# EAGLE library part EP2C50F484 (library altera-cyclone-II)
EP2C50F484 Auto generated by make-symbol-device-package-bsdl.ulp Rev. 19 Tip: Use split-device-symbol.ulp to generate a Device with multiple small symbols! Read HELP. Source: EP2C50F484.BSD
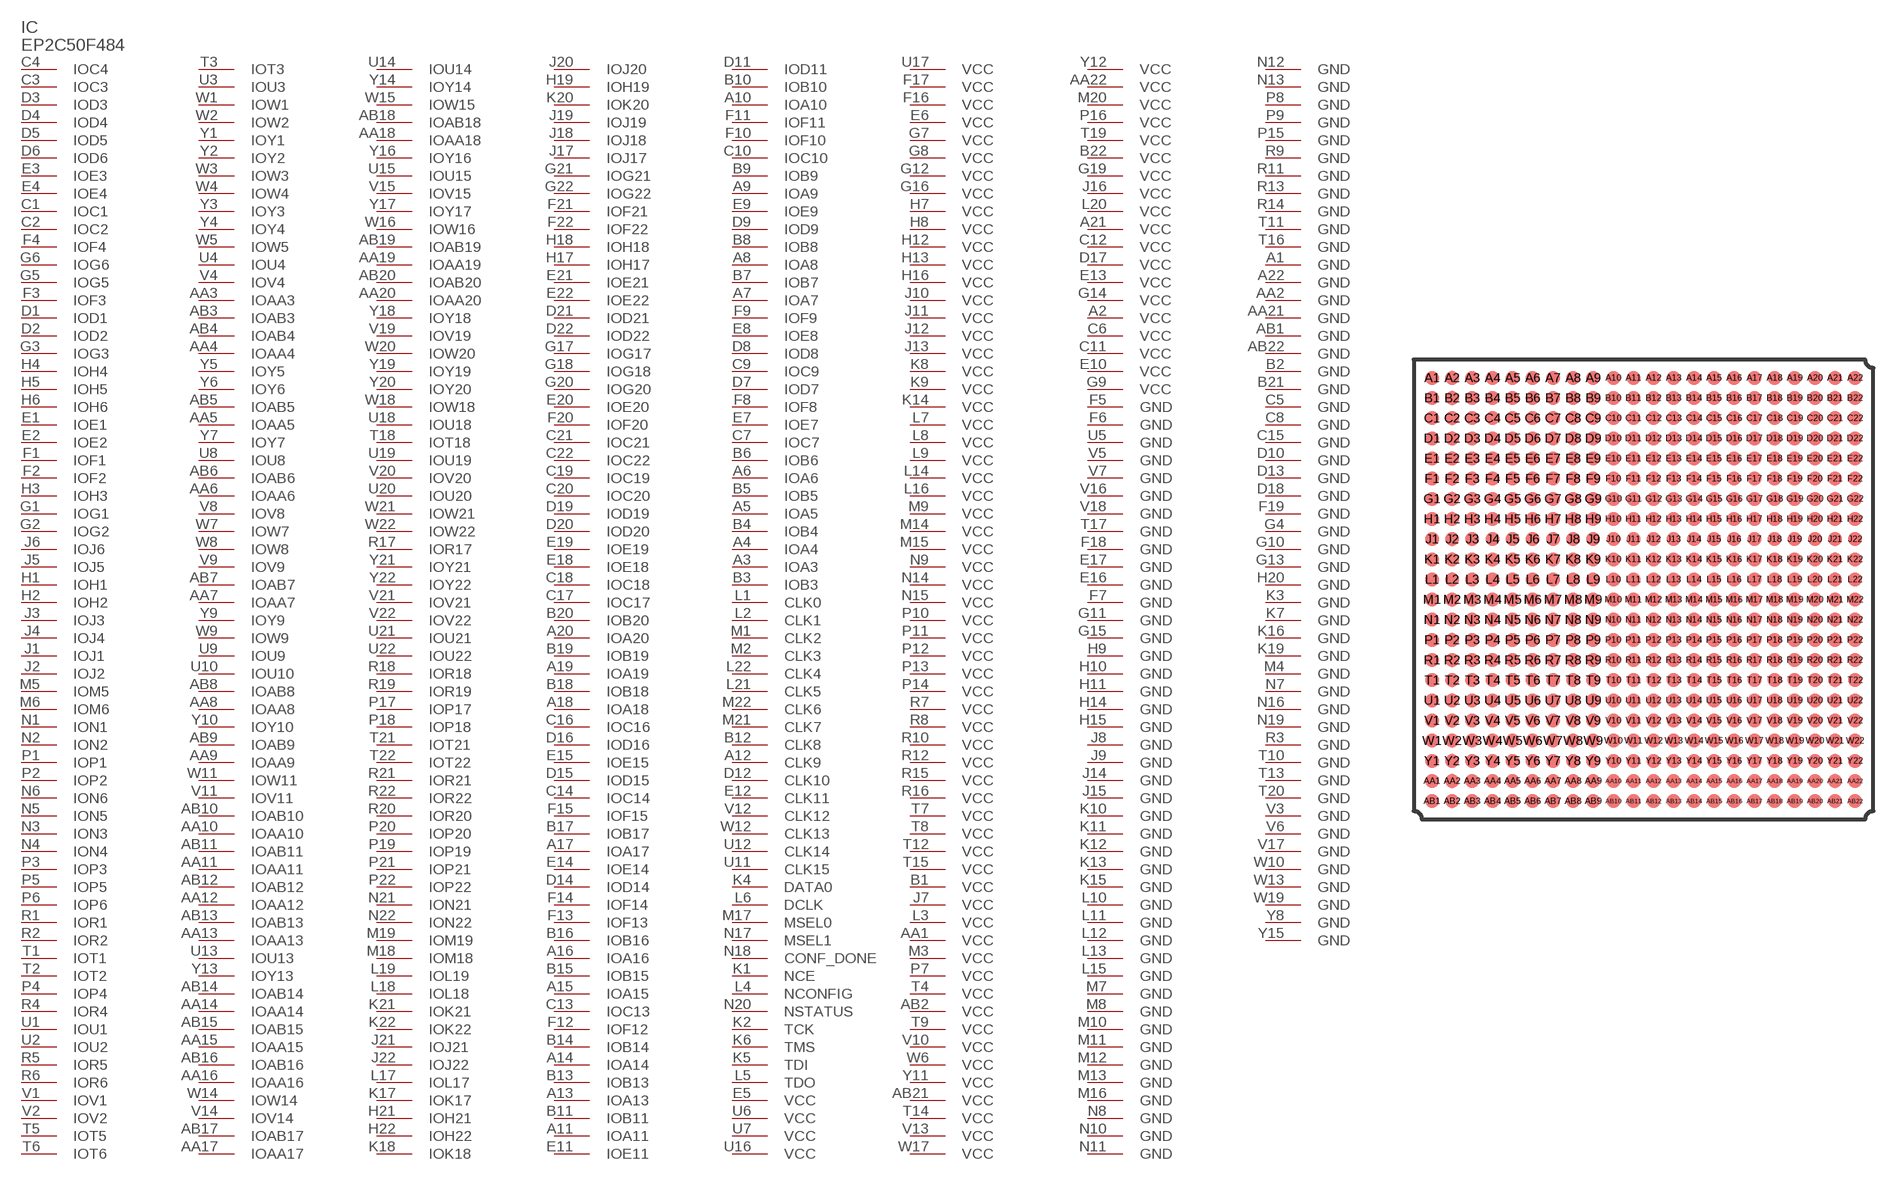
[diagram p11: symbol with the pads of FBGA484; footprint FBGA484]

Designator prefix IC

## EP2C50F484 (MPN: EP2C50F484C8N; OC_FARNELL: 1549358; OC_NEWARK: 51R0569)  [FBGA484]
A1  GND  pwr
A2  VCC  pwr
A3  IOA3
A4  IOA4
A5  IOA5
A6  IOA6
A7  IOA7
A8  IOA8
A9  IOA9
A10  IOA10
A11  IOA11
A12  CLK9
A13  IOA13
A14  IOA14
A15  IOA15
A16  IOA16
A17  IOA17
A18  IOA18
A19  IOA19
A20  IOA20
A21  VCC  pwr
A22  GND  pwr
AA1  VCC  pwr
AA2  GND  pwr
AA3  IOAA3
AA4  IOAA4
AA5  IOAA5
AA6  IOAA6
AA7  IOAA7
AA8  IOAA8
AA9  IOAA9
AA10  IOAA10
AA11  IOAA11
AA12  IOAA12
AA13  IOAA13
AA14  IOAA14
AA15  IOAA15
AA16  IOAA16
AA17  IOAA17
AA18  IOAA18
AA19  IOAA19
AA20  IOAA20
AA21  GND  pwr
AA22  VCC  pwr
AB1  GND  pwr
AB2  VCC  pwr
AB3  IOAB3
AB4  IOAB4
AB5  IOAB5
AB6  IOAB6
AB7  IOAB7
AB8  IOAB8
AB9  IOAB9
AB10  IOAB10
AB11  IOAB11
AB12  IOAB12
AB13  IOAB13
AB14  IOAB14
AB15  IOAB15
AB16  IOAB16
AB17  IOAB17
AB18  IOAB18
AB19  IOAB19
AB20  IOAB20
AB21  VCC  pwr
AB22  GND  pwr
B1  VCC  pwr
B2  GND  pwr
B3  IOB3
B4  IOB4
B5  IOB5
B6  IOB6
B7  IOB7
B8  IOB8
B9  IOB9
B10  IOB10
B11  IOB11
B12  CLK8
B13  IOB13
B14  IOB14
B15  IOB15
B16  IOB16
B17  IOB17
B18  IOB18
B19  IOB19
B20  IOB20
B21  GND  pwr
B22  VCC  pwr
C1  IOC1
C2  IOC2
C3  IOC3  out
C4  IOC4  out
C5  GND  pwr
C6  VCC  pwr
C7  IOC7
C8  GND  pwr
C9  IOC9
C10  IOC10
C11  VCC  pwr
C12  VCC  pwr
C13  IOC13
C14  IOC14
C15  GND  pwr
C16  IOC16
C17  IOC17
C18  IOC18
C19  IOC19
C20  IOC20
C21  IOC21
C22  IOC22
D1  IOD1
D2  IOD2
D3  IOD3
D4  IOD4
D5  IOD5
D6  IOD6
D7  IOD7
D8  IOD8
D9  IOD9
D10  GND  pwr
D11  IOD11
D12  CLK10
D13  GND  pwr
D14  IOD14
D15  IOD15
D16  IOD16
D17  VCC  pwr
D18  GND  pwr
D19  IOD19
D20  IOD20
D21  IOD21
D22  IOD22
E1  IOE1
E2  IOE2
E3  IOE3
E4  IOE4
E5  VCC  pwr
E6  VCC  pwr
E7  IOE7
E8  IOE8
E9  IOE9
E10  VCC  pwr
E11  IOE11
E12  CLK11
E13  VCC  pwr
E14  IOE14
E15  IOE15
E16  GND  pwr
E17  GND  pwr
E18  IOE18
E19  IOE19
E20  IOE20
E21  IOE21
E22  IOE22
F1  IOF1
F2  IOF2
F3  IOF3
F4  IOF4
F5  GND  pwr
F6  GND  pwr
F7  GND  pwr
F8  IOF8
F9  IOF9
F10  IOF10
F11  IOF11
F12  IOF12
F13  IOF13
F14  IOF14
F15  IOF15
F16  VCC  pwr
F17  VCC  pwr
F18  GND  pwr
F19  GND  pwr
F20  IOF20
F21  IOF21
F22  IOF22
G1  IOG1
G2  IOG2
G3  IOG3
G4  GND  pwr
G5  IOG5
G6  IOG6
G7  VCC  pwr
G8  VCC  pwr
G9  VCC  pwr
G10  GND  pwr
G11  GND  pwr
G12  VCC  pwr
G13  GND  pwr
G14  VCC  pwr
G15  GND  pwr
G16  VCC  pwr
G17  IOG17
G18  IOG18
G19  VCC  pwr
G20  IOG20
G21  IOG21
G22  IOG22
H1  IOH1
H2  IOH2
H3  IOH3
H4  IOH4
H5  IOH5
H6  IOH6
H7  VCC  pwr
H8  VCC  pwr
H9  GND  pwr
H10  GND  pwr
H11  GND  pwr
H12  VCC  pwr
H13  VCC  pwr
H14  GND  pwr
H15  GND  pwr
H16  VCC  pwr
H17  IOH17
H18  IOH18
H19  IOH19
H20  GND  pwr
H21  IOH21
H22  IOH22
J1  IOJ1
J2  IOJ2
J3  IOJ3
J4  IOJ4
J5  IOJ5
J6  IOJ6
J7  VCC  pwr
J8  GND  pwr
J9  GND  pwr
J10  VCC  pwr
J11  VCC  pwr
J12  VCC  pwr
J13  VCC  pwr
J14  GND  pwr
J15  GND  pwr
J16  VCC  pwr
J17  IOJ17
J18  IOJ18
J19  IOJ19
J20  IOJ20
J21  IOJ21
J22  IOJ22
K1  NCE  in
K2  TCK  in
K3  GND  pwr
K4  DATA0
K5  TDI  in
K6  TMS  in
K7  GND  pwr
K8  VCC  pwr
K9  VCC  pwr
K10  GND  pwr
K11  GND  pwr
K12  GND  pwr
K13  GND  pwr
K14  VCC  pwr
K15  GND  pwr
K16  GND  pwr
K17  IOK17
K18  IOK18
K19  GND  pwr
K20  IOK20
K21  IOK21
K22  IOK22
L1  CLK0
L2  CLK1
L3  VCC  pwr
L4  NCONFIG  in
L5  TDO  out
L6  DCLK
L7  VCC  pwr
L8  VCC  pwr
L9  VCC  pwr
L10  GND  pwr
L11  GND  pwr
L12  GND  pwr
L13  GND  pwr
L14  VCC  pwr
L15  GND  pwr
L16  VCC  pwr
L17  IOL17
L18  IOL18
L19  IOL19
L20  VCC  pwr
L21  CLK5
L22  CLK4
M1  CLK2
M2  CLK3
M3  VCC  pwr
M4  GND  pwr
M5  IOM5
M6  IOM6
M7  GND  pwr
M8  GND  pwr
M9  VCC  pwr
M10  GND  pwr
M11  GND  pwr
M12  GND  pwr
M13  GND  pwr
M14  VCC  pwr
M15  VCC  pwr
M16  GND  pwr
M17  MSEL0  in
M18  IOM18
M19  IOM19
M20  VCC  pwr
M21  CLK7
M22  CLK6
N1  ION1
N2  ION2
N3  ION3
N4  ION4
N5  ION5
N6  ION6
N7  GND  pwr
N8  GND  pwr
N9  VCC  pwr
N10  GND  pwr
N11  GND  pwr
N12  GND  pwr
N13  GND  pwr
N14  VCC  pwr
N15  VCC  pwr
N16  GND  pwr
N17  MSEL1  in
N18  CONF_DONE  in
N19  GND  pwr
N20  NSTATUS  in
N21  ION21
N22  ION22
P1  IOP1
P2  IOP2
P3  IOP3
P4  IOP4
P5  IOP5
P6  IOP6
P7  VCC  pwr
P8  GND  pwr
P9  GND  pwr
P10  VCC  pwr
P11  VCC  pwr
P12  VCC  pwr
P13  VCC  pwr
P14  VCC  pwr
P15  GND  pwr
P16  VCC  pwr
P17  IOP17
P18  IOP18
P19  IOP19
P20  IOP20
P21  IOP21
P22  IOP22
R1  IOR1
R2  IOR2
R3  GND  pwr
R4  IOR4
R5  IOR5
R6  IOR6
R7  VCC  pwr
R8  VCC  pwr
R9  GND  pwr
R10  VCC  pwr
R11  GND  pwr
R12  VCC  pwr
R13  GND  pwr
R14  GND  pwr
R15  VCC  pwr
R16  VCC  pwr
R17  IOR17
R18  IOR18
R19  IOR19
R20  IOR20
R21  IOR21
R22  IOR22
T1  IOT1
T2  IOT2
T3  IOT3
T4  VCC  pwr
T5  IOT5
T6  IOT6
T7  VCC  pwr
T8  VCC  pwr
T9  VCC  pwr
T10  GND  pwr
T11  GND  pwr
T12  VCC  pwr
T13  GND  pwr
T14  VCC  pwr
T15  VCC  pwr
T16  GND  pwr
T17  GND  pwr
T18  IOT18
T19  VCC  pwr
T20  GND  pwr
T21  IOT21
T22  IOT22
U1  IOU1
U2  IOU2
U3  IOU3
U4  IOU4
U5  GND  pwr
U6  VCC  pwr
U7  VCC  pwr
U8  IOU8
U9  IOU9
U10  IOU10
U11  CLK15
U12  CLK14
U13  IOU13
U14  IOU14
U15  IOU15
U16  VCC  pwr
U17  VCC  pwr
U18  IOU18
U19  IOU19
U20  IOU20
U21  IOU21
U22  IOU22
V1  IOV1
V2  IOV2
V3  GND  pwr
V4  IOV4
V5  GND  pwr
V6  GND  pwr
V7  GND  pwr
V8  IOV8
V9  IOV9
V10  VCC  pwr
V11  IOV11
V12  CLK12
V13  VCC  pwr
V14  IOV14
V15  IOV15
V16  GND  pwr
V17  GND  pwr
V18  GND  pwr
V19  IOV19
V20  IOV20
V21  IOV21
V22  IOV22
W1  IOW1
W2  IOW2
W3  IOW3
W4  IOW4
W5  IOW5
W6  VCC  pwr
W7  IOW7
W8  IOW8
W9  IOW9
W10  GND  pwr
W11  IOW11
W12  CLK13
W13  GND  pwr
W14  IOW14
W15  IOW15
W16  IOW16
W17  VCC  pwr
W18  IOW18
W19  GND  pwr
W20  IOW20
W21  IOW21
W22  IOW22
Y1  IOY1
Y2  IOY2
Y3  IOY3
Y4  IOY4
Y5  IOY5
Y6  IOY6
Y7  IOY7
Y8  GND  pwr
Y9  IOY9
Y10  IOY10
Y11  VCC  pwr
Y12  VCC  pwr
Y13  IOY13
Y14  IOY14
Y15  GND  pwr
Y16  IOY16
Y17  IOY17
Y18  IOY18
Y19  IOY19
Y20  IOY20
Y21  IOY21
Y22  IOY22

## Footprint FBGA484 (pad centres in mm)
EP2C15AF484 Auto generated by make-symbol-device-package-bsdl.ulp Rev. 18 Source: EP2C15AF484.BSD www.altera.com .. cyc2_cii51015.pdf
smd 0.7 x 0.7: A1 -10.5,10.5; A2 -9.5,10.5; A3 -8.5,10.5; A4 -7.5,10.5; A5 -6.5,10.5; A6 -5.5,10.5; A7 -4.5,10.5; A8 -3.5,10.5; A9 -2.5,10.5; A10 -1.5,10.5; A11 -0.5,10.5; A12 0.5,10.5; A13 1.5,10.5; A14 2.5,10.5; A15 3.5,10.5; A16 4.5,10.5; A17 5.5,10.5; A18 6.5,10.5; A19 7.5,10.5; A20 8.5,10.5; A21 9.5,10.5; A22 10.5,10.5; AA1 -10.5,-9.5; AA2 -9.5,-9.5; AA3 -8.5,-9.5; AA4 -7.5,-9.5; AA5 -6.5,-9.5; AA6 -5.5,-9.5; AA7 -4.5,-9.5; AA8 -3.5,-9.5; AA9 -2.5,-9.5; AA10 -1.5,-9.5; AA11 -0.5,-9.5; AA12 0.5,-9.5; AA13 1.5,-9.5; AA14 2.5,-9.5; AA15 3.5,-9.5; AA16 4.5,-9.5; AA17 5.5,-9.5; AA18 6.5,-9.5; AA19 7.5,-9.5; AA20 8.5,-9.5; AA21 9.5,-9.5; AA22 10.5,-9.5; AB1 -10.5,-10.5; AB2 -9.5,-10.5; AB3 -8.5,-10.5; AB4 -7.5,-10.5; AB5 -6.5,-10.5; AB6 -5.5,-10.5; AB7 -4.5,-10.5; AB8 -3.5,-10.5; AB9 -2.5,-10.5; AB10 -1.5,-10.5; AB11 -0.5,-10.5; AB12 0.5,-10.5; AB13 1.5,-10.5; AB14 2.5,-10.5; AB15 3.5,-10.5; AB16 4.5,-10.5; AB17 5.5,-10.5; AB18 6.5,-10.5; AB19 7.5,-10.5; AB20 8.5,-10.5; AB21 9.5,-10.5; AB22 10.5,-10.5; B1 -10.5,9.5; B2 -9.5,9.5; B3 -8.5,9.5; B4 -7.5,9.5; B5 -6.5,9.5; B6 -5.5,9.5; B7 -4.5,9.5; B8 -3.5,9.5; B9 -2.5,9.5; B10 -1.5,9.5; B11 -0.5,9.5; B12 0.5,9.5; B13 1.5,9.5; B14 2.5,9.5; B15 3.5,9.5; B16 4.5,9.5; B17 5.5,9.5; B18 6.5,9.5; B19 7.5,9.5; B20 8.5,9.5; B21 9.5,9.5; B22 10.5,9.5; C1 -10.5,8.5; C2 -9.5,8.5; C3 -8.5,8.5; C4 -7.5,8.5; C5 -6.5,8.5; C6 -5.5,8.5; C7 -4.5,8.5; C8 -3.5,8.5; C9 -2.5,8.5; C10 -1.5,8.5; C11 -0.5,8.5; C12 0.5,8.5; C13 1.5,8.5; C14 2.5,8.5; C15 3.5,8.5; C16 4.5,8.5; C17 5.5,8.5; C18 6.5,8.5; C19 7.5,8.5; C20 8.5,8.5; C21 9.5,8.5; C22 10.5,8.5; D1 -10.5,7.5; D2 -9.5,7.5; D3 -8.5,7.5; D4 -7.5,7.5; D5 -6.5,7.5; D6 -5.5,7.5; D7 -4.5,7.5; D8 -3.5,7.5; D9 -2.5,7.5; D10 -1.5,7.5; D11 -0.5,7.5; D12 0.5,7.5; D13 1.5,7.5; D14 2.5,7.5; D15 3.5,7.5; D16 4.5,7.5; D17 5.5,7.5; D18 6.5,7.5; D19 7.5,7.5; D20 8.5,7.5; D21 9.5,7.5; D22 10.5,7.5; E1 -10.5,6.5; E2 -9.5,6.5; E3 -8.5,6.5; E4 -7.5,6.5; E5 -6.5,6.5; E6 -5.5,6.5; E7 -4.5,6.5; E8 -3.5,6.5; E9 -2.5,6.5; E10 -1.5,6.5; E11 -0.5,6.5; E12 0.5,6.5; E13 1.5,6.5; E14 2.5,6.5; E15 3.5,6.5; E16 4.5,6.5; E17 5.5,6.5; E18 6.5,6.5; E19 7.5,6.5; E20 8.5,6.5; E21 9.5,6.5; E22 10.5,6.5; F1 -10.5,5.5; F2 -9.5,5.5; F3 -8.5,5.5; F4 -7.5,5.5; F5 -6.5,5.5; F6 -5.5,5.5; F7 -4.5,5.5; F8 -3.5,5.5; F9 -2.5,5.5; F10 -1.5,5.5; F11 -0.5,5.5; F12 0.5,5.5; F13 1.5,5.5; F14 2.5,5.5; F15 3.5,5.5; F16 4.5,5.5; F17 5.5,5.5; F18 6.5,5.5; F19 7.5,5.5; F20 8.5,5.5; F21 9.5,5.5; F22 10.5,5.5; G1 -10.5,4.5; G2 -9.5,4.5; G3 -8.5,4.5; G4 -7.5,4.5; G5 -6.5,4.5; G6 -5.5,4.5; G7 -4.5,4.5; G8 -3.5,4.5; G9 -2.5,4.5; G10 -1.5,4.5; G11 -0.5,4.5; G12 0.5,4.5; G13 1.5,4.5; G14 2.5,4.5; G15 3.5,4.5; G16 4.5,4.5; G17 5.5,4.5; G18 6.5,4.5; G19 7.5,4.5; G20 8.5,4.5; G21 9.5,4.5; G22 10.5,4.5; H1 -10.5,3.5; H2 -9.5,3.5; H3 -8.5,3.5; H4 -7.5,3.5; H5 -6.5,3.5; H6 -5.5,3.5; H7 -4.5,3.5; H8 -3.5,3.5; H9 -2.5,3.5; H10 -1.5,3.5; H11 -0.5,3.5; H12 0.5,3.5; H13 1.5,3.5; H14 2.5,3.5; H15 3.5,3.5; H16 4.5,3.5; H17 5.5,3.5; H18 6.5,3.5; H19 7.5,3.5; H20 8.5,3.5; H21 9.5,3.5; H22 10.5,3.5; J1 -10.5,2.5; J2 -9.5,2.5; J3 -8.5,2.5; J4 -7.5,2.5; J5 -6.5,2.5; J6 -5.5,2.5; J7 -4.5,2.5; J8 -3.5,2.5; J9 -2.5,2.5; J10 -1.5,2.5; J11 -0.5,2.5; J12 0.5,2.5; J13 1.5,2.5; J14 2.5,2.5; J15 3.5,2.5; J16 4.5,2.5; J17 5.5,2.5; J18 6.5,2.5; J19 7.5,2.5; J20 8.5,2.5; J21 9.5,2.5; J22 10.5,2.5; K1 -10.5,1.5; K2 -9.5,1.5; K3 -8.5,1.5; K4 -7.5,1.5; K5 -6.5,1.5; K6 -5.5,1.5; K7 -4.5,1.5; K8 -3.5,1.5; K9 -2.5,1.5; K10 -1.5,1.5; K11 -0.5,1.5; K12 0.5,1.5; K13 1.5,1.5; K14 2.5,1.5; K15 3.5,1.5; K16 4.5,1.5; K17 5.5,1.5; K18 6.5,1.5; K19 7.5,1.5; K20 8.5,1.5; K21 9.5,1.5; K22 10.5,1.5; L1 -10.5,0.5; L2 -9.5,0.5; L3 -8.5,0.5; L4 -7.5,0.5; L5 -6.5,0.5; L6 -5.5,0.5; L7 -4.5,0.5; L8 -3.5,0.5; L9 -2.5,0.5; L10 -1.5,0.5; L11 -0.5,0.5; L12 0.5,0.5; L13 1.5,0.5; L14 2.5,0.5; L15 3.5,0.5; L16 4.5,0.5; L17 5.5,0.5; L18 6.5,0.5; L19 7.5,0.5; L20 8.5,0.5; L21 9.5,0.5; L22 10.5,0.5; M1 -10.5,-0.5; M2 -9.5,-0.5; M3 -8.5,-0.5; M4 -7.5,-0.5; M5 -6.5,-0.5; M6 -5.5,-0.5; M7 -4.5,-0.5; M8 -3.5,-0.5; M9 -2.5,-0.5; M10 -1.5,-0.5; M11 -0.5,-0.5; M12 0.5,-0.5; M13 1.5,-0.5; M14 2.5,-0.5; M15 3.5,-0.5; M16 4.5,-0.5; M17 5.5,-0.5; M18 6.5,-0.5; M19 7.5,-0.5; M20 8.5,-0.5; M21 9.5,-0.5; M22 10.5,-0.5; N1 -10.5,-1.5; N2 -9.5,-1.5; N3 -8.5,-1.5; N4 -7.5,-1.5; N5 -6.5,-1.5; N6 -5.5,-1.5; N7 -4.5,-1.5; N8 -3.5,-1.5; N9 -2.5,-1.5; N10 -1.5,-1.5; N11 -0.5,-1.5; N12 0.5,-1.5; N13 1.5,-1.5; N14 2.5,-1.5; N15 3.5,-1.5; N16 4.5,-1.5; N17 5.5,-1.5; N18 6.5,-1.5; N19 7.5,-1.5; N20 8.5,-1.5; N21 9.5,-1.5; N22 10.5,-1.5; P1 -10.5,-2.5; P2 -9.5,-2.5; P3 -8.5,-2.5; P4 -7.5,-2.5; P5 -6.5,-2.5; P6 -5.5,-2.5; P7 -4.5,-2.5; P8 -3.5,-2.5; P9 -2.5,-2.5; P10 -1.5,-2.5; P11 -0.5,-2.5; P12 0.5,-2.5; P13 1.5,-2.5; P14 2.5,-2.5; P15 3.5,-2.5; P16 4.5,-2.5; P17 5.5,-2.5; P18 6.5,-2.5; P19 7.5,-2.5; P20 8.5,-2.5; P21 9.5,-2.5; P22 10.5,-2.5; R1 -10.5,-3.5; R2 -9.5,-3.5; R3 -8.5,-3.5; R4 -7.5,-3.5; R5 -6.5,-3.5; R6 -5.5,-3.5; R7 -4.5,-3.5; R8 -3.5,-3.5; R9 -2.5,-3.5; R10 -1.5,-3.5; R11 -0.5,-3.5; R12 0.5,-3.5; R13 1.5,-3.5; R14 2.5,-3.5; R15 3.5,-3.5; R16 4.5,-3.5; R17 5.5,-3.5; R18 6.5,-3.5; R19 7.5,-3.5; R20 8.5,-3.5; R21 9.5,-3.5; R22 10.5,-3.5; T1 -10.5,-4.5; T2 -9.5,-4.5; T3 -8.5,-4.5; T4 -7.5,-4.5; T5 -6.5,-4.5; T6 -5.5,-4.5; T7 -4.5,-4.5; T8 -3.5,-4.5; T9 -2.5,-4.5; T10 -1.5,-4.5; T11 -0.5,-4.5; T12 0.5,-4.5; T13 1.5,-4.5; T14 2.5,-4.5; T15 3.5,-4.5; T16 4.5,-4.5; T17 5.5,-4.5; T18 6.5,-4.5; T19 7.5,-4.5; T20 8.5,-4.5; T21 9.5,-4.5; T22 10.5,-4.5; U1 -10.5,-5.5; U2 -9.5,-5.5; U3 -8.5,-5.5; U4 -7.5,-5.5; U5 -6.5,-5.5; U6 -5.5,-5.5; U7 -4.5,-5.5; U8 -3.5,-5.5; U9 -2.5,-5.5; U10 -1.5,-5.5; U11 -0.5,-5.5; U12 0.5,-5.5; U13 1.5,-5.5; U14 2.5,-5.5; U15 3.5,-5.5; U16 4.5,-5.5; U17 5.5,-5.5; U18 6.5,-5.5; U19 7.5,-5.5; U20 8.5,-5.5; U21 9.5,-5.5; U22 10.5,-5.5; V1 -10.5,-6.5; V2 -9.5,-6.5; V3 -8.5,-6.5; V4 -7.5,-6.5; V5 -6.5,-6.5; V6 -5.5,-6.5; V7 -4.5,-6.5; V8 -3.5,-6.5; V9 -2.5,-6.5; V10 -1.5,-6.5; V11 -0.5,-6.5; V12 0.5,-6.5; V13 1.5,-6.5; V14 2.5,-6.5; V15 3.5,-6.5; V16 4.5,-6.5; V17 5.5,-6.5; V18 6.5,-6.5; V19 7.5,-6.5; V20 8.5,-6.5; V21 9.5,-6.5; V22 10.5,-6.5; W1 -10.5,-7.5; W2 -9.5,-7.5; W3 -8.5,-7.5; W4 -7.5,-7.5; W5 -6.5,-7.5; W6 -5.5,-7.5; W7 -4.5,-7.5; W8 -3.5,-7.5; W9 -2.5,-7.5; W10 -1.5,-7.5; W11 -0.5,-7.5; W12 0.5,-7.5; W13 1.5,-7.5; W14 2.5,-7.5; W15 3.5,-7.5; W16 4.5,-7.5; W17 5.5,-7.5; W18 6.5,-7.5; W19 7.5,-7.5; W20 8.5,-7.5; W21 9.5,-7.5; W22 10.5,-7.5; Y1 -10.5,-8.5; Y2 -9.5,-8.5; Y3 -8.5,-8.5; Y4 -7.5,-8.5; Y5 -6.5,-8.5; Y6 -5.5,-8.5; Y7 -4.5,-8.5; Y8 -3.5,-8.5; Y9 -2.5,-8.5; Y10 -1.5,-8.5; Y11 -0.5,-8.5; Y12 0.5,-8.5; Y13 1.5,-8.5; Y14 2.5,-8.5; Y15 3.5,-8.5; Y16 4.5,-8.5; Y17 5.5,-8.5; Y18 6.5,-8.5; Y19 7.5,-8.5; Y20 8.5,-8.5; Y21 9.5,-8.5; Y22 10.5,-8.5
